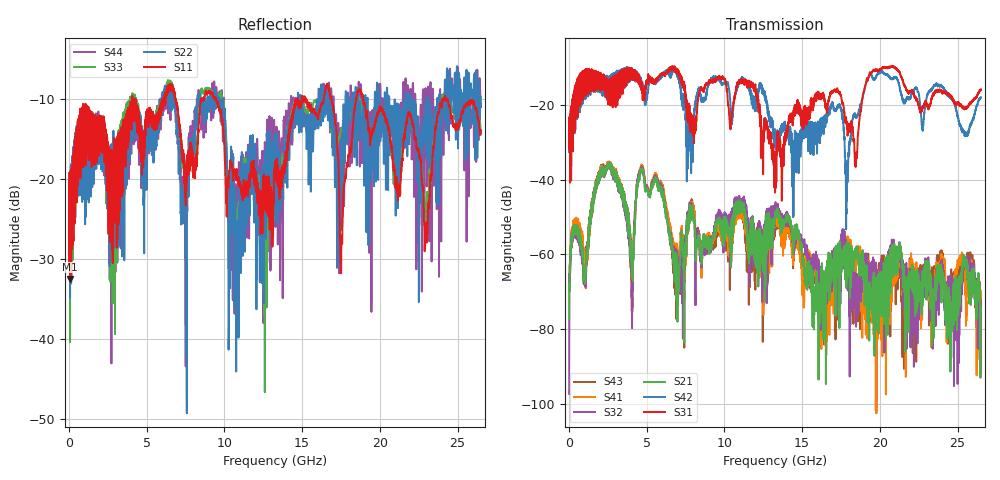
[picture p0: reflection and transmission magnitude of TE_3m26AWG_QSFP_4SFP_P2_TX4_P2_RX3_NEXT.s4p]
!Agilent Technologies,N5222A,MY51421691,A.10.00.00
!Agilent N5222A: A.10.00.00
!Date: Friday, January 30, 2015 12:36:00
!Correction: S11(Full 4 Port(1,2,3,4))
!S12(Full 4 Port(1,2,3,4))
!S13(Full 4 Port(1,2,3,4))
!S14(Full 4 Port(1,2,3,4))
!S21(Full 4 Port(1,2,3,4))
!S22(Full 4 Port(1,2,3,4))
!S23(Full 4 Port(1,2,3,4))
!S24(Full 4 Port(1,2,3,4))
!S31(Full 4 Port(1,2,3,4))
!S32(Full 4 Port(1,2,3,4))
!S33(Full 4 Port(1,2,3,4))
!S34(Full 4 Port(1,2,3,4))
!S41(Full 4 Port(1,2,3,4))
!S42(Full 4 Port(1,2,3,4))
!S43(Full 4 Port(1,2,3,4))
!S44(Full 4 Port(1,2,3,4))
!S4P File: Measurements: <S11,S12,S13,S14>,
!<S21,S22,S23,S24>,
!<S31,S32,S33,S34>,
!<S41,S42,S43,S44>:
# Hz S  dB  R 50.0
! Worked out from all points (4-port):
!   2650 points, 10 MHz to 26.5 GHz, reference 50 ohm
!   strongest paths, dB at 10 MHz, 6.63 GHz, 13.26 GHz, 19.88 GHz, 26.5 GHz:
!     S31: -24.9, -10.5, -43.4, -10.4, -15.7
!     S42: -25.1, -11.0, -28.9, -11.4, -17.8
!     S21: -77.2, -57.8, -49.8, -71.8, -74.1
!     S32: -97.4, -56.9, -48.6, -69.3, -74.7
!     S41: -66.5, -54.7, -51.4, -66.6, -76.8
!     S43: -65.9, -59.6, -50.8, -68.6, -71.0
!   lowest |S11| = -32.5 dB at 70 MHz (marker M1), VSWR 1.05, Z = 52.4 + j0.247 ohm
!   |S11| at or under -10 dB: start of sweep to 4.075 GHz; 9.454 GHz to 14.73 GHz (5.275 GHz wide, 43.6 % of centre); 18.91 GHz to 24.02 GHz (5.109 GHz wide, 23.8 % of centre)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
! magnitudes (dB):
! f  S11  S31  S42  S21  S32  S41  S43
! 10 MHz  -19.3  -24.9  -25.1  -77.2  -97.4  -66.5  -65.9
! 70 MHz  -32.5  -40.8  -37.7  -65.1  -65.0  -64.3  -65.1
! 2.6 GHz  -16.7  -13.4  -12.2  -36.7  -37.1  -36.5  -36.5
! 4.04 GHz  -10.3  -10.1  -10.6  -63.7  -69.3  -68.7  -75.2
! 4.68 GHz  -14.0  -13.9  -13.6  -37.6  -37.0  -36.7  -36.4
! 7.02 GHz  -11.9  -11.0  -11.5  -73.7  -64.7  -63.5  -69.2
! 26.5 GHz  -14.0  -15.7  -17.8  -74.1  -74.7  -76.8  -71.0
